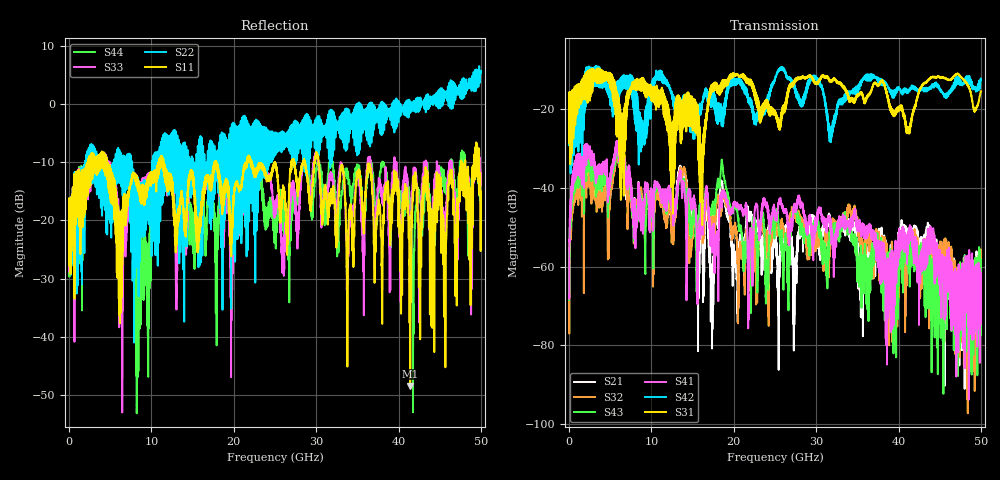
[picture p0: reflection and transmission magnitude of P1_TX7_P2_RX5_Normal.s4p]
!Keysight Technologies,N5225B,MY57041031,A.13.20.10
!Date: Friday, May 31, 2019 11:35:33
!Correction: S11(Full 4 Port(1,2,3,4))
!S12(Full 4 Port(1,2,3,4))
!S13(Full 4 Port(1,2,3,4))
!S14(Full 4 Port(1,2,3,4))
!S21(Full 4 Port(1,2,3,4))
!S22(Full 4 Port(1,2,3,4))
!S23(Full 4 Port(1,2,3,4))
!S24(Full 4 Port(1,2,3,4))
!S31(Full 4 Port(1,2,3,4))
!S32(Full 4 Port(1,2,3,4))
!S33(Full 4 Port(1,2,3,4))
!S34(Full 4 Port(1,2,3,4))
!S41(Full 4 Port(1,2,3,4))
!S42(Full 4 Port(1,2,3,4))
!S43(Full 4 Port(1,2,3,4))
!S44(Full 4 Port(1,2,3,4))
!S4P File: Measurements: <S11,S12,S13,S14>,
!<S21,S22,S23,S24>,
!<S31,S32,S33,S34>,
!<S41,S42,S43,S44>:
# Hz S  dB  R 50.0
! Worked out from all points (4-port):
!   5000 points, 10 MHz to 50 GHz, reference 50 ohm
!   strongest paths, dB at 10 MHz, 12.51 GHz, 25.01 GHz, 37.51 GHz, 50 GHz:
!     S31: -19.4, -39.5, -20.8, -14.0, -15.5
!     S42: -19.5, -17.3, -12.2, -12.7, -12.5
!     S41: -67.2, -45.9, -46.1, -54.0, -66.3
!     S43: -68.5, -45.1, -48.8, -56.1, -58.2
!     S32: -64.4, -53.1, -47.3, -51.8, -68.0
!     S21: -61.0, -49.1, -52.9, -53.0, -67.3
!   lowest |S11| = -48.4 dB at 41.42 GHz (marker M1), VSWR 1.01, Z = 49.8 - j0.319 ohm
!   |S11| at or under -10 dB: 4.612 GHz to 10.91 GHz (6.297 GHz wide, 81.1 % of centre); 11.46 GHz to 17.73 GHz (6.277 GHz wide, 43 % of centre); 30.28 GHz to 47.61 GHz (17.32 GHz wide, 44.5 % of centre)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
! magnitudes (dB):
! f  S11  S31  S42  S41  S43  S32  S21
! 10 MHz  -19.3  -19.4  -19.5  -67.2  -68.5  -64.4  -61.0
! 6.47 GHz  -22.2  -23.2  -12.5  -30.6  -30.7  -30.7  -30.6
! 17.31 GHz  -13.8  -14.3  -17.2  -52.3  -45.6  -49.2  -69.1
! 18.52 GHz  -14.8  -14.3  -22.6  -43.1  -33.2  -44.2  -38.3
! 20.37 GHz  -13.3  -11.2  -13.7  -44.1  -45.7  -53.4  -62.9
! 41.42 GHz  -48.4  -24.3  -14.6  -50.5  -55.2  -52.8  -53.2
! 50 GHz  -15.0  -15.5  -12.5  -66.3  -58.2  -68.0  -67.3
